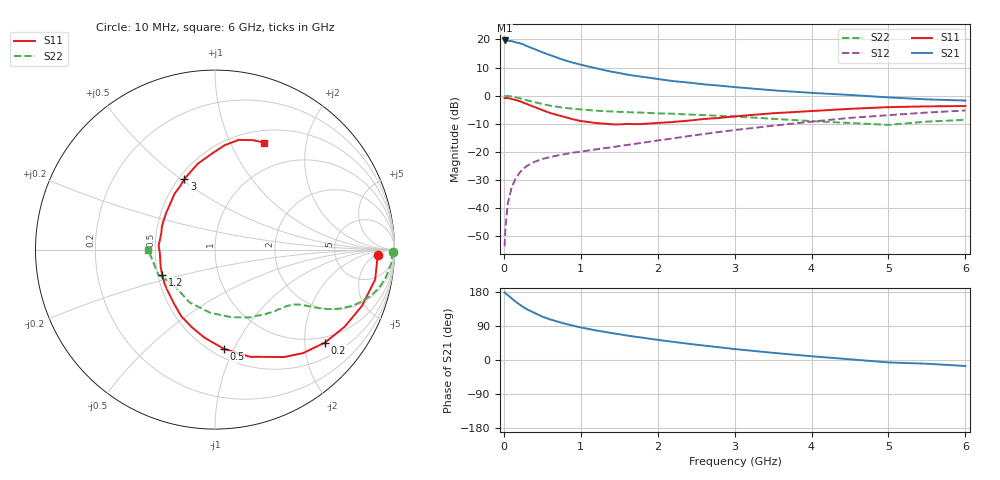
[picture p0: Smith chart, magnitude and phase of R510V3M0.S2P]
! SIEMENS Small Signal Semiconductors
! BFR183
! Si NPN RF Bipolar Junction Transistor in SOT23
! VCE = 10 V  IC = 3 mA
! Common Emitter S-Parameters:  May  1996
# GHz  S  MA  R  50
!  f  S11  S21  S12  S22
! GHz  MAG  ANG  MAG  ANG  MAG  ANG  MAG  ANG
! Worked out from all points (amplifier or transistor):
!   36 points, 10 MHz to 6 GHz, reference 50 ohm
!   highest |S21| = 19.7 dB at 10 MHz (marker M1)
!   |S21| within 3 dB of that: start of sweep to 391 MHz
!   unconditionally stable (mu >= 1): 1.293 GHz to 2.833 GHz
!   at 250 MHz: K = 0.29, MSG = 22.2 dB, |S12| = -26.1 dB
!   at 1.4 GHz: K = 1.04, MAG = 12.3 dB, |S12| = -18.4 dB
!   at 6 GHz: K = 0.87, MSG = 1.8 dB, |S12| = -5.3 dB
!   S11 on the Smith chart (normalised r, x): 10 MHz: 18, -7; 200 MHz: 0.85, -2.48; 500 MHz: 0.57, -0.91; 1.2 GHz: 0.53, -0.17; 3 GHz: 0.54, +0.51; 6 GHz: 0.64, +1.34
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0.01  0.9086 -2.0  9.614 178.3  0.0021 85.2  0.9918 -0.8
0.02  0.9053 -4.4  9.447 176.3  0.0043 87.2  0.9874 -1.8
0.05  0.9078 -10.6  9.463 171.4  0.0118 83.5  0.9848 -4.5
0.1  0.8766 -21.0  9.394 163.1  0.0229 78.3  0.9652 -9.0
0.15  0.841 -30.6  8.915 154.4  0.033 72.8  0.939 -13.1
0.2  0.8025 -40.2  8.637 147.1  0.0418 69.1  0.9068 -16.4
0.25  0.7568 -49.7  8.207 140.0  0.0497 64.4  0.8666 -19.5
0.3  0.7112 -57.3  7.632 133.9  0.0563 61.3  0.8302 -22.1
0.4  0.6283 -71.9  6.73 124.0  0.0668 56.3  0.7675 -25.4
0.5  0.5544 -85.0  5.932 114.5  0.0747 53.1  0.7109 -27.8
0.6  0.4932 -97.0  5.282 107.3  0.081 51.3  0.6649 -29.4
0.8  0.4155 -117.0  4.231 95.6  0.0915 49.3  0.6052 -31.3
0.9  0.3796 -126.7  3.861 90.5  0.097 49.3  0.5862 -32.0
1.1  0.3398 -145.6  3.305 82.0  0.1059 50.2  0.5543 -33.6
1.2  0.3262 -154.5  3.076 78.0  0.1108 50.7  0.5414 -34.4
1.6  0.3148 176.0  2.378 64.6  0.1325 52.9  0.5087 -38.2
2.2  0.3408 142.7  1.817 47.9  0.174 54.7  0.4776 -46.4
3  0.428 113.6  1.423 28.9  0.2449 52.2  0.4263 -62.4
3.5  0.4872 101.5  1.246 18.9  0.2919 48.1  0.388 -76.3
4.5  0.5835 84.8  1.03 1.9  0.4031 37.4  0.3268 -115.7
5.5  0.6456 70.8  0.86 -9.8  0.501 24.5  0.3457 -156.4
6  0.6547 65.6  0.819 -15.8  0.5462 16.1  0.3717 -179.8
